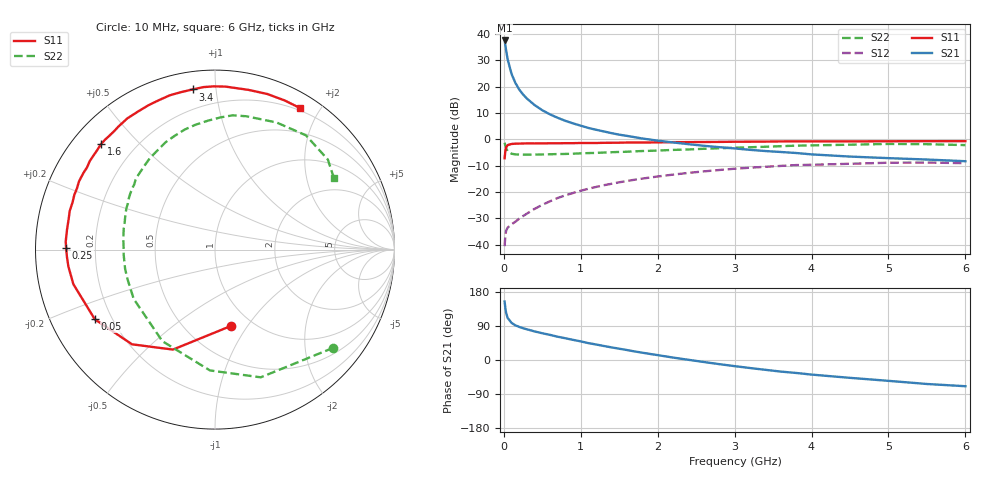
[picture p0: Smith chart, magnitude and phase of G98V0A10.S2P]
! SIEMENS Small Signal Semiconductors
! BFG235
! Si NPN RF Bipolar Junction Transistor in SOT223
! VCE = 8 V  IC = 100 mA
! Common Emitter S-Parameters:  July  1994
# GHz  S  MA  R  50
!  f  S11  S21  S12  S22
! GHz  MAG  ANG  MAG  ANG  MAG  ANG  MAG  ANG
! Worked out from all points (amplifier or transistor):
!   40 points, 10 MHz to 6 GHz, reference 50 ohm
!   highest |S21| = 37.5 dB at 10 MHz (marker M1)
!   |S21| within 3 dB of that: start of sweep to 25.72 MHz
!   unconditionally stable (mu >= 1): 480.9 MHz to 1.44 GHz
!   at 200 MHz: K = 0.76, MSG = 24.5 dB, |S12| = -30.2 dB
!   at 1.5 GHz: K = 1.00, MSG = 9.1 dB, |S12| = -16.4 dB
!   at 6 GHz: K = 0.89, MSG = 0.4 dB, |S12| = -9.1 dB
!   S11 on the Smith chart (normalised r, x): 10 MHz: 0.80, -0.84; 50 MHz: 0.14, -0.26; 250 MHz: 0.09, +0.01; 1.6 GHz: 0.08, +0.39; 3.4 GHz: 0.09, +0.87; 6 GHz: 0.17, +1.76
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0.01  0.4347 -78.3  75.11 154.3  0.0093 66.1  0.8565 -39.7
0.02  0.6042 -112.8  60.43 136.0  0.0149 50.3  0.7559 -70.3
0.03  0.7015 -131.2  48.31 124.0  0.0183 42.7  0.6738 -92.4
0.05  0.774 -149.9  32.68 110.9  0.021 34.6  0.5886 -119.9
0.1  0.8124 -166.3  17.42 97.9  0.0242 34.4  0.5297 -148.8
0.15  0.8224 -173.5  11.72 91.5  0.0271 39.9  0.5147 -161.1
0.2  0.826 -177.3  8.785 87.3  0.031 44.2  0.5121 -168.0
0.25  0.8298 179.2  7.076 83.8  0.0347 48.3  0.5092 -172.6
0.3  0.8329 176.9  5.912 81.0  0.0386 50.8  0.5096 -176.5
0.4  0.8319 172.2  4.447 75.4  0.0476 54.2  0.5096 178.2
0.5  0.8328 168.4  3.549 70.6  0.0567 55.8  0.5135 173.9
0.6  0.8375 165.1  2.964 66.3  0.0663 56.4  0.5176 170.1
0.7  0.8362 161.6  2.552 61.4  0.0765 56.4  0.5223 166.7
0.9  0.8414 156.1  1.997 53.1  0.0952 54.3  0.5311 160.6
1.1  0.8485 149.7  1.636 44.5  0.1146 51.4  0.545 154.7
1.6  0.8652 137.2  1.157 26.3  0.1608 41.9  0.5781 141.1
2.2  0.8792 123.8  0.868 6.4  0.2127 29.2  0.626 125.3
3.2  0.8975 102.2  0.628 -21.2  0.2876 6.1  0.7036 99.0
3.4  0.901 97.9  0.596 -25.9  0.2995 1.3  0.7192 93.2
4.5  0.9092 78.2  0.468 -47.1  0.3417 -24.0  0.7869 64.2
5.5  0.9173 64.9  0.411 -63.3  0.3607 -46.2  0.8044 38.6
6  0.92 58.9  0.382 -69.2  0.3506 -54.6  0.773 30.9
